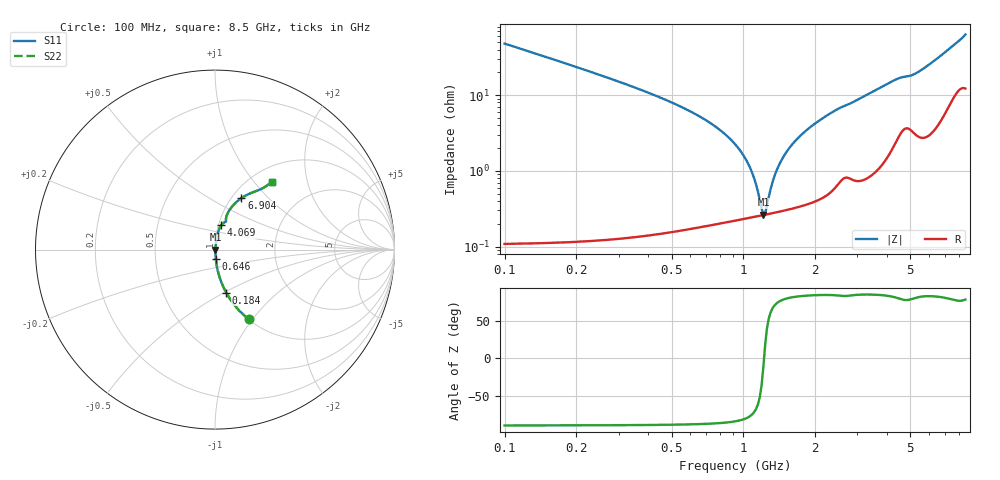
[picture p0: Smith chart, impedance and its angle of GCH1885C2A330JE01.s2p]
!Murata Part Number: GCH1885C2A330JE01
!These Parameters are Measured in Series Mode Connection
!Data Generated on Jun 19, 2026
!  o--ll--o
!Port1  Port2
!  o------o
!Operation Temp=25[degC], DC Bias Voltage=0[V]
!Freq. Start=100[MHz] Stop=9[GHz] 401[Steps]
# Hz S RI R 50
!Freq.(Hz) S11(Real) S11(Imag) S21(Real) S21(Imag) S12(Real) S12(Imag) S22(Real) S22(Imag)
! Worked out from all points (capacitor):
!   401 points, 100 MHz to 8.5 GHz, reference 50 ohm
!   read as one part in series: C = 33 pF near 142 MHz
!   lowest |Z| = 264 mohm at 1.213 GHz (marker M1)
!   series resonance near 1.22 GHz, so ESL is about 520 pH
!   S11 on the Smith chart (normalised r, x): 100 MHz: 1.00, -0.96; 184 MHz: 1.00, -0.51; 646 MHz: 1.00, -0.11; 4.069 GHz: 1.03, +0.29; 6.904 GHz: 1.11, +0.71; 8.5 GHz: 1.24, +1.24
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1e8  0.1872 -0.3889  0.8128 0.3889  0.8128 0.3889  0.1872 -0.3889
1.84e8  0.0625 -0.2398  0.9375 0.2398  0.9375 0.2398  0.0625 -0.2398
3.52e8  0.0168 -0.1232  0.9832 0.1232  0.9832 0.1232  0.0168 -0.1232
6.46e8  0.00462 -0.0533  0.9954 0.0533  0.9954 0.0533  0.00462 -0.0533
8.56e8  0.0029 -0.0284  0.9971 0.0284  0.9971 0.0284  0.0029 -0.0284
1.003e9  0.00255 -0.0155  0.9975 0.0155  0.9975 0.0155  0.00255 -0.0155
1.087e9  0.0025 -0.00911  0.9975 0.00911  0.9975 0.00911  0.0025 -0.00911
1.171e9  0.00255 -0.00323  0.9975 0.00323  0.9975 0.00323  0.00255 -0.00323
1.213e9  0.0026 -0.00045  0.9974 0.00045  0.9974 0.00045  0.0026 -0.00045
1.255e9  0.00266 0.00224  0.9973 -0.00224  0.9973 -0.00224  0.00266 0.00224
1.381e9  0.00293 0.00986  0.9971 -0.00986  0.9971 -0.00986  0.00293 0.00986
1.507e9  0.0033 0.0169  0.9967 -0.0169  0.9967 -0.0169  0.0033 0.0169
1.717e9  0.00412 0.0279  0.9959 -0.0279  0.9959 -0.0279  0.00412 0.0279
2.032e9  0.00589 0.0433  0.9941 -0.0433  0.9941 -0.0433  0.00589 0.0433
2.452e9  0.0102 0.0627  0.9898 -0.0627  0.9898 -0.0627  0.0102 0.0627
2.914e9  0.0139 0.0804  0.9861 -0.0804  0.9861 -0.0804  0.0139 0.0804
4.069e9  0.0352 0.1363  0.9648 -0.1363  0.9648 -0.1363  0.0352 0.1363
4.3e9  0.0442 0.1463  0.9558 -0.1463  0.9558 -0.1463  0.0442 0.1463
5.707e9  0.0713 0.2039  0.9287 -0.2039  0.9287 -0.2039  0.0713 0.2039
6.904e9  0.1466 0.2864  0.8534 -0.2864  0.8534 -0.2864  0.1466 0.2864
7.114e9  0.1665 0.2987  0.8335 -0.2987  0.8335 -0.2987  0.1665 0.2987
8.5e9  0.3172 0.3772  0.6828 -0.3772  0.6828 -0.3772  0.3172 0.3772
